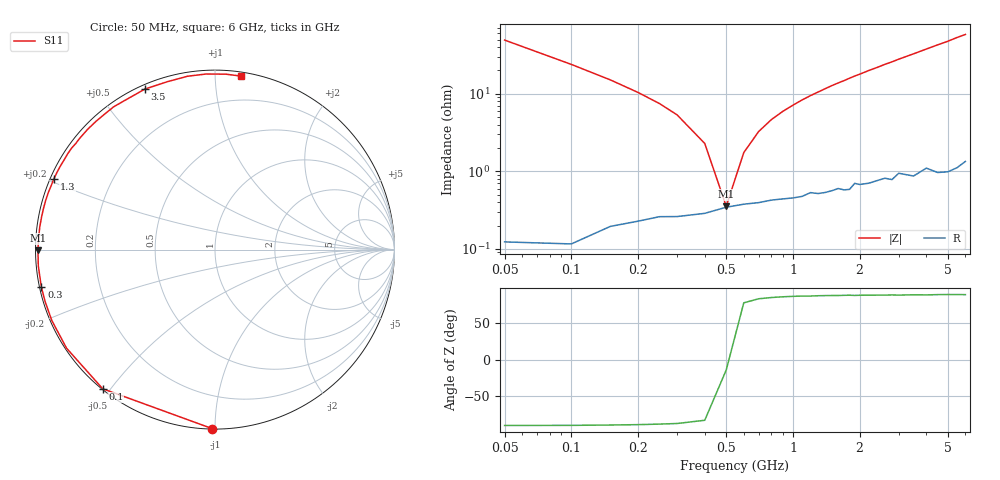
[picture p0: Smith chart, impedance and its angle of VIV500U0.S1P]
! Infineon Technologies  Discrete & RF Semiconductors
! BB 804
! Si Tuning Diode in SOT23
! VR = 0.5 V
! S-Parameters:  July  1999
# GHz  S  MA  R  50
!  f  S11
! GHz  MAG  ANG
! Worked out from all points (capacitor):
!   34 points, 50 MHz to 6 GHz, reference 50 ohm
!   read as one part to ground: C = 64 pF near 50 MHz
!   lowest |Z| = 356 mohm at 500 MHz (marker M1)
!   series resonance near 504.9 MHz, so ESL is about 1.6 nH
!   S11 on the Smith chart (normalised r, x): 50 MHz: 0.00, -0.98; 100 MHz: 0.00, -0.48; 300 MHz: 0.01, -0.11; 1.3 GHz: 0.01, +0.21; 3.5 GHz: 0.02, +0.65; 6 GHz: 0.03, +1.16
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0.05  0.9975 -90.9
0.1  0.9962 -128.9
0.15  0.9929 -146.4
0.2  0.9913 -156.5
0.25  0.9899 -163.0
0.3  0.9897 -167.8
0.4  0.9886 -174.8
0.5  0.9863 -179.8
0.6  0.985 176.1
0.8  0.9832 169.4
1.1  0.9817 161.1
1.3  0.9804 156.2
1.5  0.979 151.4
1.6  0.9779 149.2
1.7  0.979 147.1
1.9  0.9752 142.6
2  0.9762 140.7
2.2  0.976 136.5
2.4  0.9748 132.8
2.6  0.9738 128.8
2.8  0.9756 125.4
3  0.9716 121.7
3.5  0.9759 113.6
4  0.9724 105.9
4.5  0.9779 99.0
5  0.9795 92.9
5.5  0.9793 86.5
6  0.9774 81.4
